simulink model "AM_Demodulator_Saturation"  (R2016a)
settings: Solver=ode3  StartTime=0.0  StopTime=6  FixedStep=1/5000000  RelTol=1e-3
libraries: dsparch4 x4

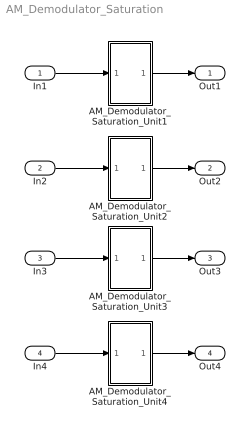
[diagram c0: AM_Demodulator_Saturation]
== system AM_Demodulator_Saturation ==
  In1 : Inport
  In2 : Inport  Port=2
  In3 : Inport  Port=3
  In4 : Inport  Port=4
  AM_Demodulator_Saturation_Unit1 : Subsystem
  AM_Demodulator_Saturation_Unit2 : Subsystem
  AM_Demodulator_Saturation_Unit3 : Subsystem
  AM_Demodulator_Saturation_Unit4 : Subsystem
  Out1 : Outport
  Out2 : Outport  Port=2
  Out3 : Outport  Port=3
  Out4 : Outport  Port=4
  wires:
  AM_Demodulator_Saturation_Unit4/1(Out1) -> Out4/1
  In3/1 -> AM_Demodulator_Saturation_Unit3/1(In)
  In4/1 -> AM_Demodulator_Saturation_Unit4/1(In)
  AM_Demodulator_Saturation_Unit3/1(Out1) -> Out3/1
  AM_Demodulator_Saturation_Unit2/1(Out1) -> Out2/1
  In2/1 -> AM_Demodulator_Saturation_Unit2/1(In)
  AM_Demodulator_Saturation_Unit1/1(Out1) -> Out1/1
  In1/1 -> AM_Demodulator_Saturation_Unit1/1(In)

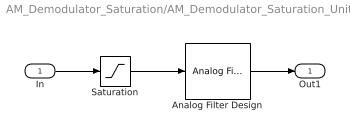
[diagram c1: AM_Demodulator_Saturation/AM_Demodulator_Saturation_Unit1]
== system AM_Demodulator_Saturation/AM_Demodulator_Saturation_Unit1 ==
  In : Inport
  Analog Filter Design : dsparch4/Analog Filter Design  method=Butterworth  filttype=Lowpass  N=8  Wlo=45000*2*pi  Whi=80  Rp=2  Rs=40
  Saturation : Saturate  UpperLimit=inf  LowerLimit=0
  Out1 : Outport
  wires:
  In/1 -> Saturation/1
  Analog Filter Design/1 -> Out1/1
  Saturation/1 -> Analog Filter Design/1

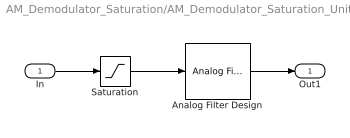
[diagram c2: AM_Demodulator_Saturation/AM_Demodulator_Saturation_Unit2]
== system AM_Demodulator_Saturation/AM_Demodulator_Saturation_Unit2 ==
  In : Inport
  Analog Filter Design : dsparch4/Analog Filter Design  method=Butterworth  filttype=Lowpass  N=8  Wlo=45000*2*pi  Whi=80  Rp=2  Rs=40
  Saturation : Saturate  UpperLimit=inf  LowerLimit=0
  Out1 : Outport
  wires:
  In/1 -> Saturation/1
  Analog Filter Design/1 -> Out1/1
  Saturation/1 -> Analog Filter Design/1

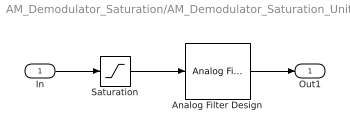
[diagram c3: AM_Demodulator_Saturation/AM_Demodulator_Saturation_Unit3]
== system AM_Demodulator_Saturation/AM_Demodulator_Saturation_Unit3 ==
  In : Inport
  Analog Filter Design : dsparch4/Analog Filter Design  method=Butterworth  filttype=Lowpass  N=8  Wlo=45000*2*pi  Whi=80  Rp=2  Rs=40
  Saturation : Saturate  UpperLimit=inf  LowerLimit=0
  Out1 : Outport
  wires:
  In/1 -> Saturation/1
  Analog Filter Design/1 -> Out1/1
  Saturation/1 -> Analog Filter Design/1

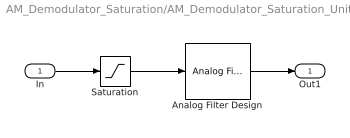
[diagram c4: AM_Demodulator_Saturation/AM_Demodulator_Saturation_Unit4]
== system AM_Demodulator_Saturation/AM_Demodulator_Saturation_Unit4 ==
  In : Inport
  Analog Filter Design : dsparch4/Analog Filter Design  method=Butterworth  filttype=Lowpass  N=8  Wlo=45000*2*pi  Whi=80  Rp=2  Rs=40
  Saturation : Saturate  UpperLimit=inf  LowerLimit=0
  Out1 : Outport
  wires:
  In/1 -> Saturation/1
  Analog Filter Design/1 -> Out1/1
  Saturation/1 -> Analog Filter Design/1
